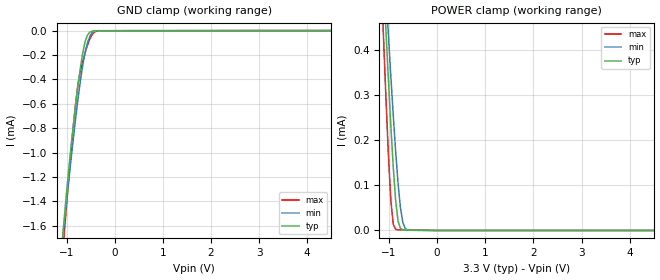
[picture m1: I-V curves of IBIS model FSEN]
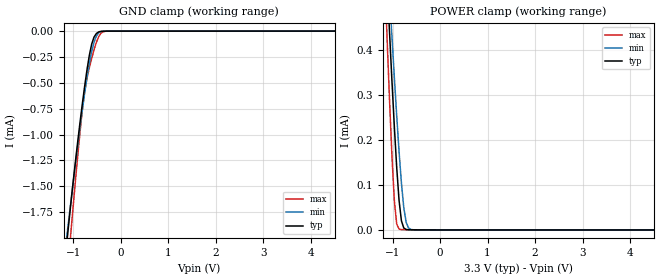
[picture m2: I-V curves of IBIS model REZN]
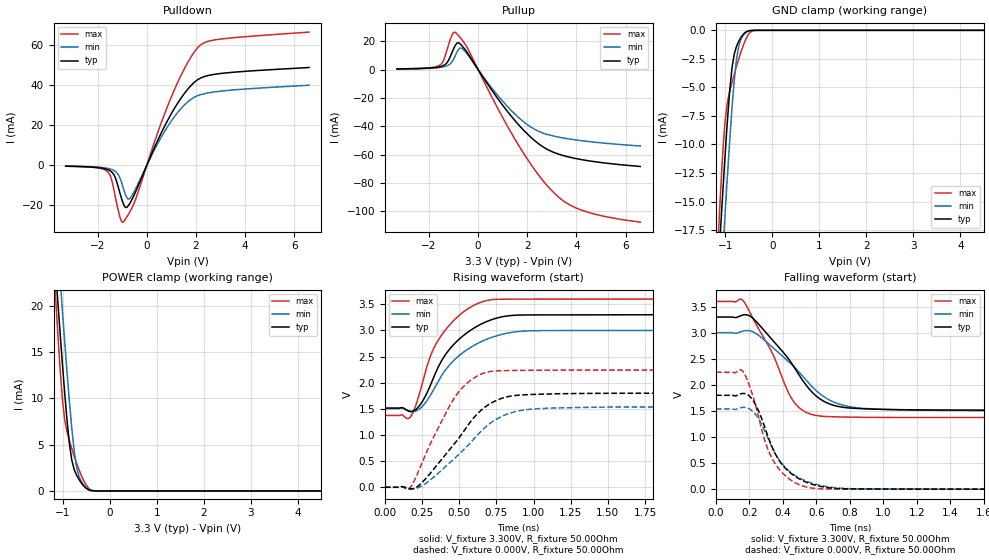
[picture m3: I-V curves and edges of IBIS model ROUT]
| Texas Instruments Incorporated
| QUAD CHANNEL M-LVDS RECEIVERS
| Marketing part#   Voltage Range   Package-type   #pins/pkg drawing
| SN65MLVD048RGZR   3.0V - 5.5V   VQFN   48-pin QFN
| SN65MLVD048RGZT   3.0V - 5.5V   VQFN   48-pin QFN/Small
[IBIS Ver]   4.0
[File name]   sn65mlvd048.ibs
[File Rev]   1.0
[Date]   03/07/2011
[Source]   Model built from TISPICE simulations at:
   Texas Instruments Incorporated.
   Analog-eLab, HPA
   12500 TI Blvd
   Dallas, TX -75243
   For Support e-mail: elab_scm_ibis@list.ti.com
[Notes]   Revision History
   Rev 1.0: 03/07/2011
   - Model based on simulations from TIspice
   - ccomp values are based on PVT conditions although listed
   in numerical order, please review ccomp comments below under
   respective [Model]
[Disclaimer] This product is designed as an aid for customers of Texas
   Instruments.
   No warranties, either expressed or implied, with respect
   to this third party software (if any) or with respect to
   its fitness for any particular purpose is claimed by Texas
   Instruments or the author. The software (if any) is provided
   solely on an "as is" basis. The entire risk as to its quality
   and performance is with the customer
[Copyright]   (C)Copyright 2011 Texas Instruments Incorporated.
   All rights reserved.
|   Component sn65mlvd048rgz
[Component]   sn65mlvd048rgz
[Manufacturer]  Texas Instruments Incorporated
[Package]   |48-pin QFN package
|   typ   min   max
R_pkg   0.091884286   0.05095   0.10827
L_pkg   1.564798571nH   1.22682nH   1.79617nH
C_pkg   0.352638095pF   0.32567pF   0.40056pF
[Pin] signal_name   model_name   R_pin   L_pin   C_pin
1   NC   NC   0.00507   0.50436nH   0.25222pF
2   VCC   POWER   0.05453   1.44952nH   0.38679pF
3   2A   A_B_IN   0.10244   1.65488nH   0.35368pF
4   2B   A_B_IN   0.10188   1.61488nH   0.34309pF
5   NC   NC   0.004   0.37135nH   0.25645pF
6   GND   GND   0.04999   1.20252nH   0.35539pF
7   GND   GND   0.04985   1.19873nH   0.35525pF
8   NC   NC   0.004   0.3713nH   0.2565pF
9   3A   A_B_IN   0.10255   1.62476nH   0.34383pF
10   3B   A_B_IN   0.10316   1.66538nH   0.35597pF
11   VCC   POWER   0.05504   1.46605nH   0.38939pF
12   NC   NC   0.00507   0.50446nH   0.25213pF
13   4A   A_B_IN   0.10769   1.78773nH   0.33719pF
14   4B   A_B_IN   0.10651   1.7467nH   0.36884pF
15   VCC   POWER   0.05573   1.42696nH   0.40172pF
16   VCC   POWER   0.05343   1.32944nH   0.38799pF
17   NC   NC   0.00393   0.36665nH   0.25841pF
18   GND   GND   0.04971   1.19158nH   0.35341pF
19   3REN   REZN   0.09506   1.46808nH   0.32567pF
20   3FSEN   FSEN   0.09536   1.48828nH   0.33741pF
21   4REN   REZN   0.09765   1.54419nH   0.34899pF
22   4FSEN   FSEN   0.10289   1.65093nH   0.36609pF
23   GND   GND   0.05875   1.58201nH   0.41278pF
24   VCC   POWER   0.05766   1.52803nH   0.37429pF
25   NC   NC   0.00498   0.49884nH   0.25434pF
26   4R   ROUT   0.05587   1.48017nH   0.40056pF
27   GND   GND   0.05274   1.32633nH   0.39094pF
28   NC   NC   0.00423   0.39452nH   0.2666pF
29   3R   ROUT   0.05095   1.22682nH   0.36955pF
30   PDN   NC   0.09792   1.50475nH   0.33235pF
31   GND   GND   0.05157   1.22971nH   0.3603pF
32   NC   NC   0.00393   0.36665nH   0.25842pF
33   2R   ROUT   0.05366   1.32882nH   0.38pF
34   GND   GND   0.05404   1.36471nH   0.38892pF
35   NC   NC   0.00514   0.47754nH   0.28414pF
36   1R   ROUT   0.05465   1.44237nH   0.36592pF
37   VCC   POWER   0.05681   1.503nH   0.3827pF
38   GND   GND   0.05623   1.50107nH   0.41098pF
39   1FSEN   FSEN   0.09941   1.60072nH   0.36103pF
40   1REN   REZN   0.09589   1.51932nH   0.3453pF
41   2FSEN   FSEN   0.09511   1.48505nH   0.33655pF
42   2REN   REZN   0.0956   1.47617nH   0.32567pF
43   GND   GND   0.09692   1.49583nH   0.32549pF
44   NC   NC   0.09958   1.55179nH   0.34125pF
45   VCC   POWER   0.0531   1.32799nH   0.3911pF
46   VCC   POWER   0.05551   1.42116nH   0.40259pF
47   1A   A_B_IN   0.10705   1.7546nH   0.3698pF
48   1B   A_B_IN   0.10827   1.79617nH   0.33791pF
[Diff_pin]   inv_pin   vdiff   tdelay_typ   tdelay_min   tdelay_max
| The A and B are Diff_pins
3   4   NA   NA   NA   NA
9   10   NA   NA   NA   NA
13   14   NA   NA   NA   NA
47   48   NA   NA   NA   NA
| Models and submodels in the file (4): FSEN (Input), REZN (Input), ROUT (3-state), A_B_IN (Input)
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|   FSEN Model
[Model]   FSEN
Model_type   Input
Vinl   = 0.80V
Vinh   = 2.00V
|   typ   min   max
|   (nom PVT)   (Fast PVT)   (Slow PVT)
C_comp   3.3085444pF   2.9897475pF   3.5451622pF
[Voltage Range]   3.3   3.0   3.6
|Junction temperature
[Temperature Range]   37   97   -40
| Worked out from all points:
|   GND clamp passes 1 mA (typ) near -0.92 V on its own axis
|   POWER clamp passes 1 mA (typ) near -1.31 V on its own axis
|ambient temperature   25   85   -40
[GND Clamp]
|   Voltage   I(typ)   I(min)   I(max)
-3.3V     -14.29mA   -11.85mA   -18.05mA
-1.111V   -1.828mA   -1.833mA   -1.98mA
-1.061V   -1.601mA   -1.639mA   -1.731mA
-1.012V   -1.381mA   -1.448mA   -1.488mA
-912.1mV  -972.3uA   -1.077mA   -1.023mA
-812.6mV  -614.2uA   -726.8uA   -605.3uA
-762.8mV  -454.6uA   -564.2uA   -441.4uA
-663.3mV  -184uA     -284.4uA   -252.2uA
-613.6mV  -89.85uA   -178.8uA   -182uA
-464.3mV  -4.577uA   -15.36uA   -29.76uA
-265.3mV  -1.132uA   -683.8nA   -2.082uA
6.6V      0A         0A         0A
[POWER Clamp]
|   Voltage   I(typ)   I(min)   I(max)
-3.3V     5.863mA    5.098mA    7.125mA
-1.161V   658.2uA    711.2uA    556.5uA
-1.111V   546.3uA    615.8uA    418.1uA
-1.061V   436.8uA    521.9uA    285.8uA
-1.012V   331uA      429.8uA    164.5uA
-961.8mV  230.8uA    340.5uA    66.31uA
-912.1mV  139.9uA    254.9uA    14.01uA
-862.3mV  66.11uA    175.1uA    2.737uA
-762.8mV  4.782uA    49.96uA    1.323uA
-713.1mV  1.427uA    17.37uA    1.227uA
-613.6mV  683.4nA    1.397uA    1.051uA
6.6V      0A         0A         0A
|   REZN Model
[Model]   REZN
Model_type   Input
Vinl   = 0.80V
Vinh   = 2.00V
|   typ   min   max
|   (nom PVT)   (Fast PVT)   (Slow PVT)
C_comp   3.2932859pF   2.9623446pF   3.5288326pF
[Voltage Range]   3.3   3.0   3.6
|Junction temperature
[Temperature Range]   37   97   -40
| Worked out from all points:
|   GND clamp passes 1 mA (typ) near -0.89 V on its own axis
|   POWER clamp passes 1 mA (typ) near -1.31 V on its own axis
|ambient temperature   25   85   -40
[GND Clamp]
|   Voltage   I(typ)   I(min)   I(max)
-3.3V     -14.35mA   -11.89mA   -18.12mA
-1.161V   -2.154mA   -2.078mA   -2.543mA
-1.111V   -1.927mA   -1.881mA   -2.269mA
-1.061V   -1.706mA   -1.687mA   -2mA
-1.012V   -1.493mA   -1.496mA   -1.736mA
-812.6mV  -711.9uA   -770.8uA   -770uA
-713.1mV  -377.2uA   -450.9uA   -454.6uA
-613.6mV  -126uA     -196uA     -263.8uA
-563.8mV  -57.74uA   -107.3uA   -180.4uA
-464.3mV  -7.66uA    -15.89uA   -52.02uA
-265.3mV  -576.9nA   -362.9nA   -1.112uA
6.6V      0A         0A         0A
[POWER Clamp]
|   Voltage   I(typ)   I(min)   I(max)
-3.3V     5.863mA    5.098mA    7.125mA
-1.161V   658.2uA    711.2uA    556.4uA
-1.111V   546.2uA    615.8uA    418uA
-1.061V   436.8uA    521.8uA    285.6uA
-1.012V   330.9uA    429.8uA    164.2uA
-961.8mV  230.7uA    340.4uA    65.91uA
-912.1mV  139.8uA    254.8uA    13.35uA
-862.3mV  65.88uA    175uA      2.008uA
-762.8mV  4.385uA    49.8uA     666nA
-713.1mV  1.039uA    17.16uA    613.9nA
-613.6mV  349.4nA    1.173uA    525.4nA
6.6V      0A         0A         0A
|   ROUT MODEL
[Model]   ROUT
Model_type   3-state
Polarity   Non-Inverting
Enable   Active-Low
Vmeas   = 1.65V
Vref   = 0V
Cref   = 15pF
Rref   = 500Ohms
|3-state   typ   min   max
|   (Nom PVT)   (Fast PVT)   (Slow PVT)
C_comp   0.84751609pF   0.84049221pF 0.86126714pF
| HIGH STATE   (Nom PVT)   (Fast PVT)   (Slow PVT)
|C_comp   0.83249355pF   0.83486872pF 0.83103616pF
| LOW STATE   (Nom PVT)   (Fast PVT)   (Slow PVT)
|C_comp   0.83104843pF   0.83099688pF 0.83485957pF
[Voltage Range]   3.3   3.0   3.6
|Junction temperature
[Temperature Range]   37   97   -40
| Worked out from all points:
|   slope of the pulldown table from 0 to 0.495 V, typ, clamps not added: 35.8 ohm
|   slope of the pullup table from 0 to 0.495 V, typ, clamps not added: 38.2 ohm
|   GND clamp passes 1 mA (typ) near -0.72 V on its own axis
|   POWER clamp passes 1 mA (typ) near -0.63 V on its own axis
|   falling waveform, V_fixture 3.300V, R_fixture 50.00Ohm: 20-80 % time 256ps typ, 286ps min, 198ps max; typ from 3.3 V to 1.51 V
|   rising waveform, V_fixture 3.300V, R_fixture 50.00Ohm: 20-80 % time 252ps typ, 276ps min, 216ps max; typ from 1.51 V to 3.3 V
|   rising waveform, V_fixture 0.000V, R_fixture 50.00Ohm: 20-80 % time 302ps typ, 338ps min, 242ps max; typ from 0 V to 1.8 V
|   falling waveform, V_fixture 0.000V, R_fixture 50.00Ohm: 20-80 % time 165ps typ, 178ps min, 142ps max; typ from 1.8 V to 0 V
|ambient temperature   25   85   -40
[Pulldown]
|   Voltage   I(typ)   I(min)   I(max)
-3.3V     -458.3uA   -414.1uA   -470.5uA
-1.609V   -2.086mA   -1.515mA   -3.051mA
-1.459V   -3.039mA   -1.974mA   -6.039mA
-1.31V    -5.407mA   -2.812mA   -14.05mA
-1.061V   -15.28mA   -7.392mA   -27.16mA
-961.8mV  -19.01mA   -11.22mA   -28.46mA
-812.6mV  -21.04mA   -16.16mA   -25.86mA
-663.3mV  -18.45mA   -16.2mA    -22.68mA
928.6mV   24.3mA     20.92mA    32.14mA
2.073V    42.82mA    34.81mA    58.84mA
2.919V    45.77mA    36.96mA    62.99mA
6.6V      48.89mA    40.04mA    66.61mA
[GND Clamp]
|   Voltage   I(typ)   I(min)   I(max)
-3.3V     -187.8mA   -193.5mA   -228.3mA
-1.161V   -21.51mA   -26.99mA   -18.88mA
-1.111V   -17.97mA   -23.39mA   -14.74mA
-1.061V   -14.52mA   -19.85mA   -11.02mA
-1.012V   -11.22mA   -16.39mA   -8.102mA
-961.8mV  -8.146mA   -13.05mA   -6.372mA
-862.3mV  -3.36mA    -6.944mA   -4.603mA
-762.8mV  -1.389mA   -2.505mA   -3.144mA
-713.1mV  -934.1uA   -1.331mA   -2.464mA
-514.1mV  -49.06uA   -78.59uA   -375.8uA
-315.1mV  -158.1nA   -713.7nA   -1.27uA
6.6V      0A         0A         0A
[Pullup]
|   Voltage   I(typ)   I(min)   I(max)
-3.3V     418.1uA    390.2uA    443.2uA
-1.559V   1.933mA    1.45mA     3.074mA
-1.26V    4.885mA    2.672mA    14.06mA
-1.061V   12.01mA    5.467mA    24.28mA
-912.1mV  17.43mA    10.37mA    25.96mA
-762.8mV  18.58mA    14.79mA    23.29mA
-613.6mV  15.92mA    14.34mA    20.08mA
1.476V    -35.5mA    -31.02mA   -48.35mA
2.272V    -49.66mA   -41.84mA   -69.87mA
2.968V    -57.6mA    -46.44mA   -84.85mA
4.312V    -63.82mA   -50.4mA    -99.74mA
6.6V      -68.36mA   -53.91mA   -107.6mA
[POWER Clamp]
|   Voltage   I(typ)   I(min)   I(max)
-3.3V     190.8mA    197mA      231mA
-1.161V   24.25mA    30.28mA    21.42mA
-1.111V   20.67mA    26.65mA    17.18mA
-1.061V   17.17mA    23.06mA    13.26mA
-1.012V   13.78mA    19.54mA    9.946mA
-961.8mV  10.56mA    16.11mA    7.672mA
-862.3mV  5.135mA    9.682mA    5.432mA
-812.6mV  3.371mA    6.843mA    4.589mA
-713.1mV  1.745mA    2.704mA    3.053mA
-663.3mV  1.285mA    1.659mA    2.364mA
-464.3mV  138uA      219.1uA    355.8uA
6.6V      0A         0A         0A
[Ramp]
R_load = 50.00Ohm
|   typ   min   max
dV/dt_r   1.080V/302.288ps 923.205mV/337.955ps   1.345V/241.562ps
dV/dt_f   1.071V/256.011ps 896.208mV/286.335ps   1.336V/197.537ps
[Falling Waveform]
V_fixture = 3.300V
V_fixture_min = 3.000V
V_fixture_max = 3.600V
R_fixture = 50.00Ohm
|   Time   V(typ)   V(min)   V(max)
0s        3.3V       3V         3.6V
160ps     3.338V     3.029V     3.623V
230ps     3.248V     3.001V     3.217V
340ps     2.849V     2.714V     2.586V
450ps     2.423V     2.397V     1.748V
510ps     2.122V     2.195V     1.529V
590ps     1.81V      1.916V     1.418V
740ps     1.58V      1.626V     1.384V
950ps     1.533V     1.536V     1.376V
3.5ns     1.515V     1.506V     1.374V
[Rising Waveform]
V_fixture = 3.300V
V_fixture_min = 3.000V
V_fixture_max = 3.600V
R_fixture = 50.00Ohm
|   Time   V(typ)   V(min)   V(max)
0s        1.515V     1.506V     1.374V
170ps     1.452V     1.447V     1.336V
200ps     1.471V     1.448V     1.501V
250ps     1.629V     1.541V     1.96V
310ps     1.972V     1.773V     2.53V
370ps     2.359V     2.08V      2.861V
500ps     2.833V     2.519V     3.287V
680ps     3.164V     2.825V     3.568V
1.01ns    3.297V     2.995V     3.599V
3.5ns     3.3V       3V         3.6V
[Rising Waveform]
V_fixture = 0.000V
V_fixture_min = 0.000V
V_fixture_max = 0.000V
R_fixture = 50.00Ohm
|   Time   V(typ)   V(min)   V(max)
0s        20.39uV    25.61uV    17.08uV
170ps     -32.74mV   -26.1mV    -9.484mV
250ps     88.44mV    26.67mV    466.1mV
330ps     351.2mV    196.7mV    970.1mV
470ps     835.8mV    555.2mV    1.718V
570ps     1.23V      833.8mV    2.031V
690ps     1.566V     1.182V     2.203V
850ps     1.745V     1.425V     2.235V
1.05ns    1.781V     1.506V     2.24V
3.5ns     1.8V       1.539V     2.242V
[Falling Waveform]
V_fixture = 0.000V
V_fixture_min = 0.000V
V_fixture_max = 0.000V
R_fixture = 50.00Ohm
|   Time   V(typ)   V(min)   V(max)
0s        1.8V       1.539V     2.242V
160ps     1.835V     1.569V     2.264V
200ps     1.784V     1.539V     1.983V
240ps     1.597V     1.416V     1.566V
290ps     1.201V     1.126V     947.7mV
340ps     771.9mV    769.2mV    562mV
420ps     382.1mV    395.9mV    240.1mV
550ps     121mV      141.5mV    33.9mV
860ps     4.244mV    5.089mV    1.382mV
3.5ns     20.39uV    25.61uV    17.08uV
